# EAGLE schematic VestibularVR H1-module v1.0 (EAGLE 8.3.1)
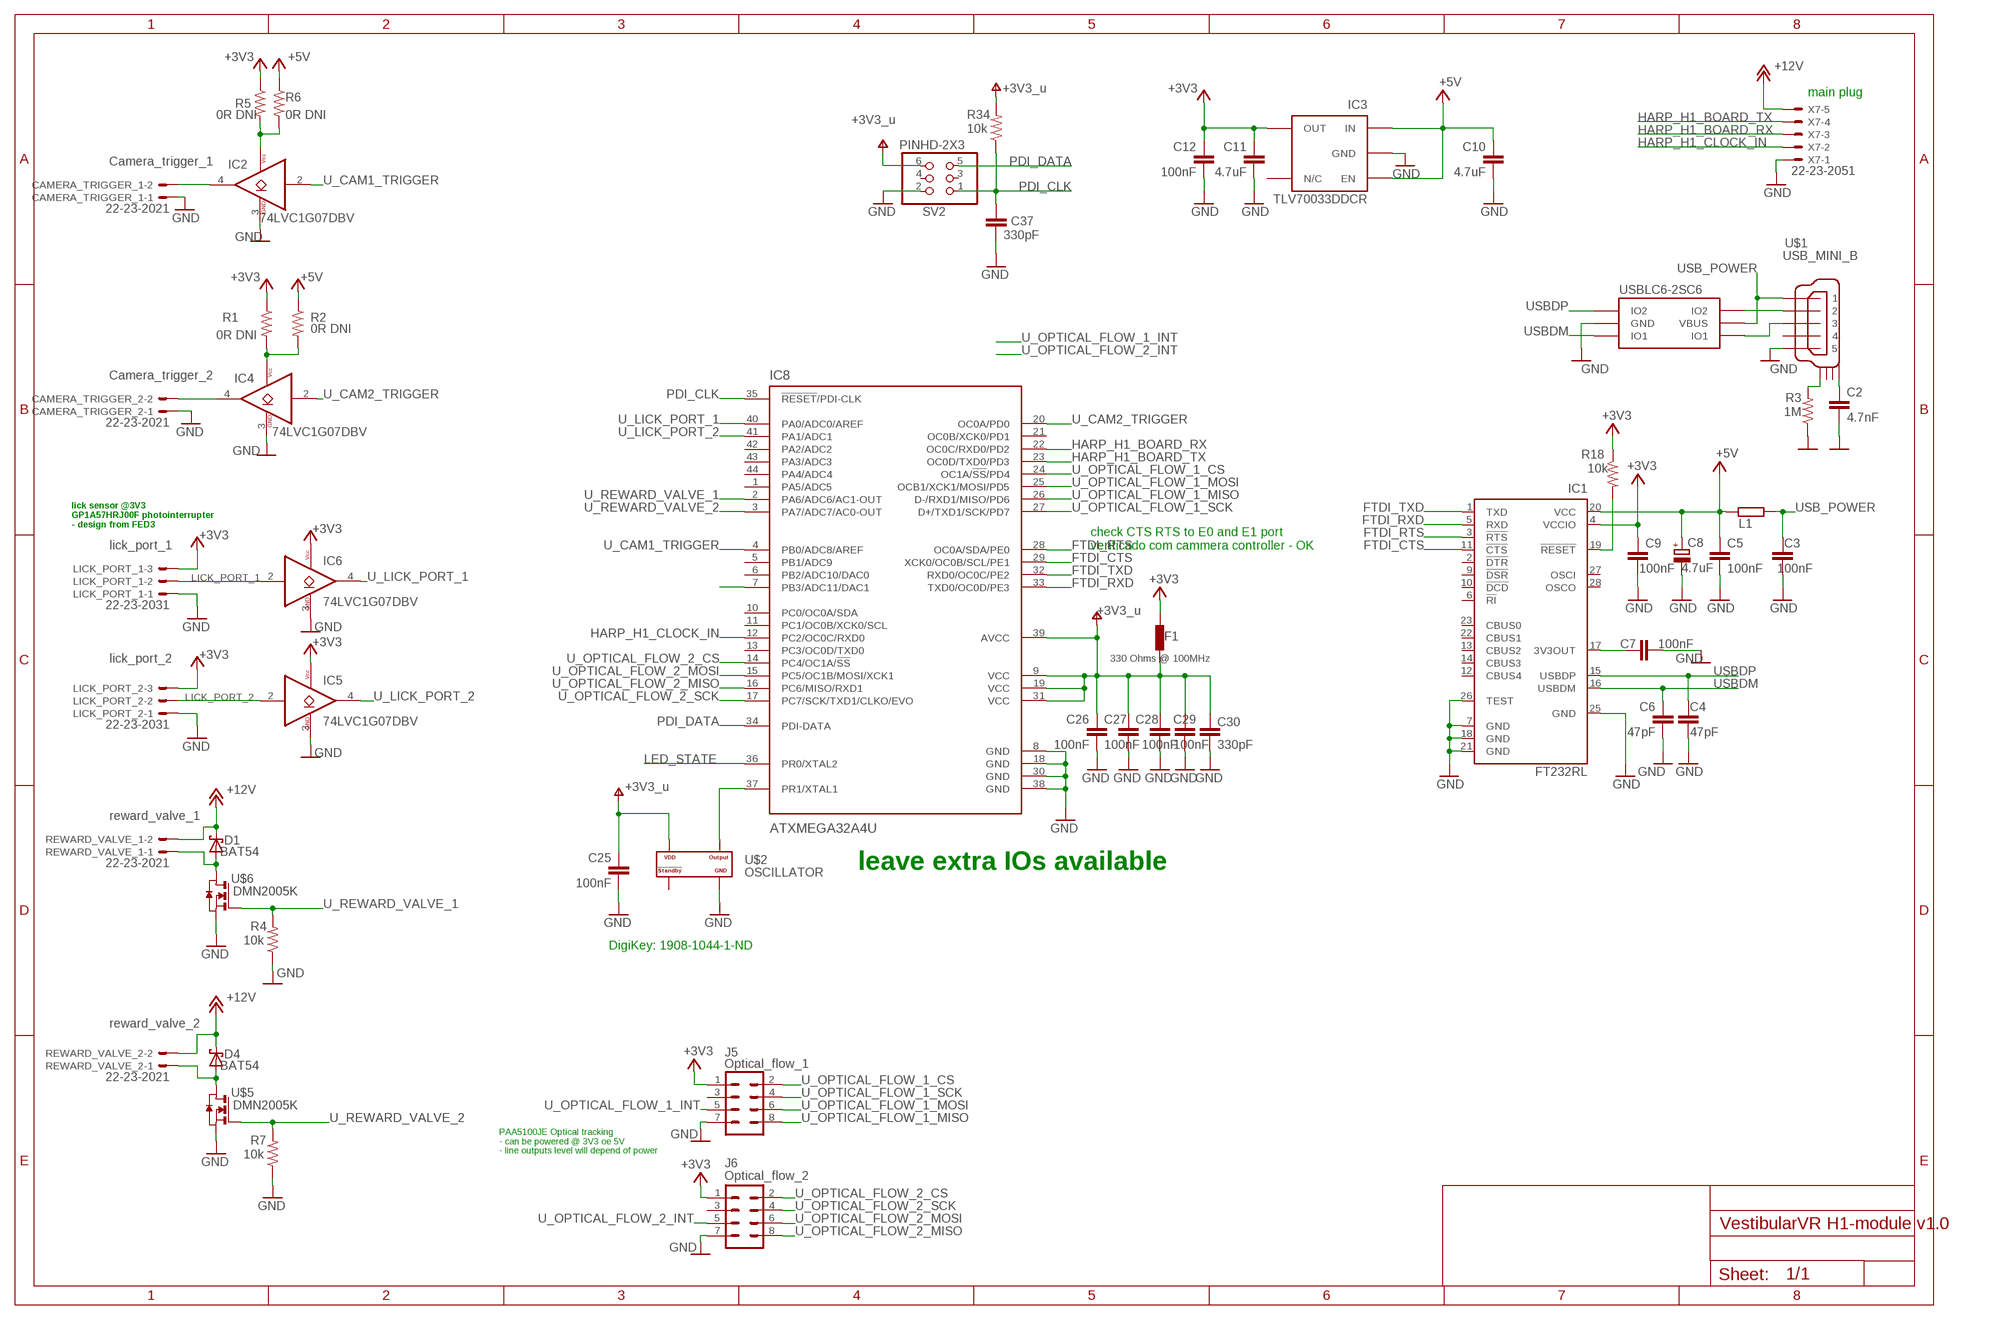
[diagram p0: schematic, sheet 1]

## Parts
C2  4.7nF  C-EUC0402  [C0402]
C3  100nF  C-EUC0402  [C0402]
C4  47pF  C-EUC0402  [C0402]
C5  100nF  C-EUC0402  [C0402]
C6  47pF  C-EUC0402  [C0402]
C7  100nF  C-EUC0402  [C0402]
C8  4.7uF  CPOL-EUA/3216-18R  [A/3216-18R]
C9  100nF  C-EUC0402  [C0402]
C10  4.7uF  C-EUC0603  [C0603]
C11  4.7uF  C-EUC0603  [C0603]
C12  100nF  C-EUC0402  [C0402]
C25  100nF  C-EUC0402  [C0402]
C26  100nF  C-EUC0402  [C0402]
C27  100nF  C-EUC0402  [C0402]
C28  100nF  C-EUC0402  [C0402]
C29  100nF  C-EUC0402  [C0402]
C30  330pF  C-EUC0402  [C0402]
C37  330pF  C-EUC0402  [C0402]
CAMERA_TRIGGER_1  22-23-2021  [22-23-2021]
CAMERA_TRIGGER_2  22-23-2021  [22-23-2021]
D1  BAT54  [SOT23]
D4  BAT54  [SOT23]
F1  330 Ohms @ 100MHz  BLM15HF0603  [R0603]
IC1  FT232RL  [SSOP28]
IC2  74LVC1G07DBV  [SOT23-5]
IC3  TLV70033DDCR  TLV700XX  [TSOT23-5]
IC4  74LVC1G07DBV  [SOT23-5]
IC5  74LVC1G07DBV  [SOT23-5]
IC6  74LVC1G07DBV  [SOT23-5]
IC7  USBLC6-2SC6  [SOT23-6L]
IC8  ATXMEGA32A4U  XMEGA-A4_AT-XMEGA-XXA4-AUTQFP44  [TQFP44]
J5  Optical_flow_1  CONN_04X2  [2X4]
J6  Optical_flow_2  CONN_04X2  [2X4]
L1  40R@100MHz  R-EU_R0805  [R0805]
LICK_PORT_1  22-23-2031  [22-23-2031]
LICK_PORT_2  22-23-2031  [22-23-2031]
R1  0R DNI  R-US_R0402  [R0402]
R2  0R DNI  R-US_R0402  [R0402]
R3  1M  R-US_R0402  [R0402]
R4  10k  R-US_R0402  [R0402]
R5  0R DNI  R-US_R0402  [R0402]
R6  0R DNI  R-US_R0402  [R0402]
R7  10k  R-US_R0402  [R0402]
R18  10k  R-US_R0402  [R0402]
R34  10k  R-US_R0402  [R0402]
REWARD_VALVE_1  22-23-2021  [22-23-2021]
REWARD_VALVE_2  22-23-2021  [22-23-2021]
SV2  PINHD-2X3  [2X03]
U$1  USB_MINI_B  [240-0002-1]
U$2  OSCILLATOR  [OSCILLATOR_3.2X2.5]
U$5  DMN2005K  [SOT23]
U$6  DMN2005K  [SOT23]
X7  22-23-2051  [22-23-2051]

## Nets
+3V3: C9.1 C11.1 C12.1 F1.2 IC1.4(VCCIO) IC3.5(OUT) IC5.5(VCC) IC6.5(VCC) J5.1 J6.1 LICK_PORT_1.3 LICK_PORT_2.3 R1.1 R5.1 R18.1
+3V3_U: C25.1 C26.1 C27.1 C28.1 C29.1 C30.1 F1.1 IC8.9(VCC) IC8.19(VCC) IC8.31(VCC) IC8.39(AVCC) R34.2 SV2.6 U$2.P$4(VDD) ; supply symbol labelled +3V3_u
+5V: C5.1 C8.+ C10.1 IC1.20(VCC) IC3.1(IN) IC3.3(EN) L1.1 R2.1 R6.1
+12V: X7.5
FTDI_CTS: IC1.11(!CTS) IC8.29(XCK0/OC0B/SCL/PE1)
FTDI_RTS: IC1.3(!RTS) IC8.28(OC0A/SDA/PE0)
FTDI_RXD: IC1.5(RXD) IC8.33(TXD0/OC0D/PE3)
FTDI_TXD: IC1.1(TXD) IC8.32(RXD0/OC0C/PE2)
GND: C2.2 C3.2 C4.2 C5.2 C6.2 C7.2 C8.- C9.2 C10.2 C11.2 C12.2 C25.2 C26.2 C27.2 C28.2 C29.2 C30.2 C37.2 CAMERA_TRIGGER_1.1 CAMERA_TRIGGER_2.1 IC1.7(GND) IC1.18(GND) IC1.21(GND) IC1.25(GND) IC1.26(TEST) IC2.3(GND) IC3.2(GND) IC4.3(GND) IC5.3(GND) IC6.3(GND) IC7.P$2(GND) IC8.8(GND) IC8.18(GND) IC8.30(GND) IC8.38(GND) J5.7 J6.7 LICK_PORT_1.1 LICK_PORT_2.1 R3.1 R4.1 R7.1 SV2.2 U$1.P$5 U$2.P$2(GND) U$5.2(S) U$6.2(S) X7.1
HARP_H1_BOARD_RX: IC8.22(OC0C/RXD0/PD2) X7.3
HARP_H1_BOARD_TX: IC8.23(OC0D/TXD0/PD3) X7.4
HARP_H1_CLOCK_IN: IC8.12(PC2/OC0C/RXD0) X7.2
LED_STATE: IC8.36(PR0/XTAL2)
LICK_PORT_1: IC6.2(A) LICK_PORT_1.2
LICK_PORT_2: IC5.2(A) LICK_PORT_2.2
N$1: R3.2 U$1.SHIELD_1
N$2: IC7.P$4(IO2) U$1.P$2
N$3: IC7.P$6(IO1) U$1.P$3
N$4: CAMERA_TRIGGER_2.2 IC4.4(Y)
N$5: IC4.5(VCC) R1.2 R2.2
N$6: D4.1(A) REWARD_VALVE_2.1 U$5.3(D)
N$7: D4.3(C) REWARD_VALVE_2.2
N$8: D1.3(C) REWARD_VALVE_1.2
N$9: D1.1(A) REWARD_VALVE_1.1 U$6.3(D)
N$14: IC2.5(VCC) R5.2 R6.2
N$16: CAMERA_TRIGGER_1.2 IC2.4(Y)
N$38: C7.1 IC1.17(3V3OUT)
N$59: C2.1 U$1.SHIELD_4
N$175: IC1.19(!RESET) R18.2
OSC2: IC8.37(PR1/XTAL1) U$2.P$3(OUTPUT)
PDI_CLK: C37.1 IC8.35(!RESET!/PDI-CLK) R34.1 SV2.1
PDI_DATA: IC8.34(PDI-DATA) SV2.5
U_CAM1_TRIGGER: IC2.2(A) IC8.4(PB0/ADC8/AREF)
U_CAM2_TRIGGER: IC4.2(A) IC8.20(OC0A/PD0)
U_HARPH1CLOCKIN: IC8.7(PB3/ADC11/DAC1)
U_LICK_PORT_1: IC6.4(Y) IC8.40(PA0/ADC0/AREF)
U_LICK_PORT_2: IC5.4(Y) IC8.41(PA1/ADC1)
U_OPTICAL_FLOW_1_CS: IC8.24(OC1A/!SS!/PD4) J5.2
U_OPTICAL_FLOW_1_INT: J5.5
U_OPTICAL_FLOW_1_MISO: IC8.26(D-/RXD1/MISO/PD6) J5.8
U_OPTICAL_FLOW_1_MOSI: IC8.25(OCB1/XCK1/MOSI/PD5) J5.6
U_OPTICAL_FLOW_1_SCK: IC8.27(D+/TXD1/SCK/PD7) J5.4
U_OPTICAL_FLOW_2_CS: IC8.14(PC4/OC1A/!SS) J6.2
U_OPTICAL_FLOW_2_INT: J6.5
U_OPTICAL_FLOW_2_MISO: IC8.16(PC6/MISO/RXD1) J6.8
U_OPTICAL_FLOW_2_MOSI: IC8.15(PC5/OC1B/MOSI/XCK1) J6.6
U_OPTICAL_FLOW_2_SCK: IC8.17(PC7/SCK/TXD1/CLKO/EVO) J6.4
U_REWARD_VALVE_1: IC8.2(PA6/ADC6/AC1-OUT) R4.2 U$6.1(G)
U_REWARD_VALVE_2: IC8.3(PA7/ADC7/AC0-OUT) R7.2 U$5.1(G)
USB_POWER: C3.1 IC7.P$5(VBUS) L1.2 U$1.P$1
USBDM: C6.1 IC1.16(USBDM) IC7.P$1(IO1)
USBDP: C4.1 IC1.15(USBDP) IC7.P$3(IO2)
Unconnected: IC1.2(!DTR) IC1.6(!RI) IC1.9(!DSR) IC1.10(!DCD) IC1.12(CBUS4) IC1.13(CBUS2) IC1.14(CBUS3) IC1.22(CBUS1) IC1.23(CBUS0) IC1.27(OSCI) IC1.28(OSCO) IC2.1(NC) IC3.4(N/C) IC4.1(NC) IC5.1(NC) IC6.1(NC) IC8.1(PA5/ADC5) IC8.5(PB1/ADC9) IC8.6(PB2/ADC10/DAC0) IC8.10(PC0/OC0A/SDA) IC8.11(PC1/OC0B/XCK0/SCL) IC8.13(PC3/OC0D/TXD0) IC8.21(OC0B/XCK0/PD1) IC8.42(PA2/ADC2) IC8.43(PA3/ADC3) IC8.44(PA4/ADC4) J5.3 J6.3 SV2.3 SV2.4 U$1.P$4 U$1.SHIELD_2 U$1.SHIELD_3 U$2.P$1(STANDBY#)

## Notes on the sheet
- main plug
- Camera_trigger_1
- Camera_trigger_2
- lick sensor @3V3
  GP1A57HRJ00F photointerrupter
  - design from FED3
- lick_port_1
- check CTS RTS to E0 and E1 port
  verificado com cammera controller - OK
- lick_port_2
- reward_valve_1
- leave extra IOs available
- DigiKey: 1908-1044-1-ND
- reward_valve_2
- PAA5100JE Optical tracking
  - can be powered @ 3V3 oe 5V
  - line outputs level will depend of power

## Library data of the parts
C2 = rcl:C-EU: CAPACITOR, European symbol; MPN: 04025C472KAT2A; SPICEPREFIX: C
C3 C5 C7 C9 = rcl:C-EU: CAPACITOR, European symbol; MPN: MC0402B104K160CT; SPICEPREFIX: C
C4 C6 = rcl:C-EU: CAPACITOR, European symbol; MPN: 04025A470JAT2A; SPICEPREFIX: C
C8 = rcl:CPOL-EU: POLARIZED CAPACITOR, European symbol; MPN: TAJA475K010; SPICEPREFIX: C
C10 C11 = rcl:C-EU: CAPACITOR, European symbol; MPN: C1608X6S1C475K080AC; NOTES: -; SPICEPREFIX: C; TYPE: SMD
C12 = rcl:C-EU: CAPACITOR, European symbol; MPN: MC0402B104K160CT; NOTES: -; SPICEPREFIX: C; TYPE: SMD
C25-C29 = rcl:C-EU: CAPACITOR, European symbol; DIGIKEY_PN: 445-5932-1-ND; MPN: C1005X7R1H104K050BB; NOTES: -; SPICEPREFIX: C; TYPE: SMD
C30 C37 = rcl:C-EU: CAPACITOR, European symbol; DIGIKEY_PN: 399-7787-1-ND; MPN: C0402C331J5GACTU; NOTES: -; SPICEPREFIX: C; TYPE: SMD
CAMERA_TRIGGER_1 CAMERA_TRIGGER_2 REWARD_VALVE_1 REWARD_VALVE_2 = con-molex:22-23-2021: .100" (2.54mm) Center Header - 2 Pin; MF: MOLEX; MPN: 22-23-2021; OC_FARNELL: 1462926; OC_NEWARK: 25C3832
D1 D4 = diode:BAT54: Schottky Diodes
F1 = VestibularVR H1-module v1.0:BLM15H: EMIFIL (R) Chip Ferrite Bead for GHz Noise; DIGIKEY_PN: 490-3997-1-ND; MOUSER_PN: 81-BLM18SG331TN1D; MPN: BLM18SG331TN1D; NOTES: -; TYPE: SMD
IC1 = VestibularVR H1-module v1.0:FT232R: UART/FIFO IC
IC2 IC4-IC6 = VestibularVR H1-module v1.0:74LVC1G07: Single Buffer/Driver With Open-Drain Output
IC3 = VestibularVR H1-module v1.0:TLV700XX: C REG LINEAR 3.3V 200MA SOT23-5; MPN: TLV70033DDCR; NOTES: -; TYPE: SMD
IC7 = VestibularVR H1-module v1.0:USBLC6-2SC6: TVS DIODE 5.25VWM 17VC SOT23-6
IC8 = VestibularVR H1-module v1.0:XMEGA-A4_AT-XMEGA-XXA4-AU: ATxMega a4 Serie; DIGIKEY_PN: ATXMEGA32A4U-AURCT-ND; MOUSER_PN: 556-ATXMEGA32A4U-AU; MPN: ATXMEGA32A4U-AUR
J5 J6 = SparkFun-Connectors:CONN_04X2: Multi connection point. Often used as Generic Header-pin footprint for 0.1 inch spaced/style header connections On any of the 0.1 inch spaced packages, you can populate with these: Break Away Headers - Straight (PRT-00116) Break Away Male Headers - Right Angle (PRT-00553) Female Headers (PRT-00115)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
L1 = rcl:R-EU_: RESISTOR, European symbol; MPN: MI0805K400R-10; SPICEPREFIX: R
LICK_PORT_1 LICK_PORT_2 = con-molex:22-23-2031: .100" (2.54mm) Center Header - 3 Pin; MF: MOLEX; MPN: 22-23-2031; OC_FARNELL: 1462950; OC_NEWARK: 30C0862
R1 R2 R5 R6 = rcl:R-US_: RESISTOR, American symbol; SPICEPREFIX: R
R3 = rcl:R-US_: RESISTOR, American symbol; PN: CRCW04021M00FKED; SPICEPREFIX: R
R4 R7 R34 = rcl:R-US_: RESISTOR, American symbol; DIGIKEY_PN: 541-3959-1-ND; MPN: CRCW040210K0FKED; NOTES: -; SPICEPREFIX: R; TYPE: SMD
R18 = rcl:R-US_: RESISTOR, American symbol; MPN: CRCW040210K0FKED; SPICEPREFIX: R
SV2 = Connector:PINHD-2X3: PIN HEADER; CATEGORY: CONNECTOR; SUB-CATEGORY: PIN-HEADER
U$1 = VestibularVR H1-module v1.0:USB_MINI_B: CONN RCPT USB2.0 MINI B SMD R/A
U$2 = VestibularVR H1-module v1.0:OSCILLATOR: XTAL OSC TCXO 32.0000MHZ HCMOS
U$5 U$6 = VestibularVR H1-module v1.0:DMN2005K: N-CHANNEL ENHANCEMENT MODE FIELD EFFECT TRANSISTOR
X7 = con-molex:22-23-2051: .100" (2.54mm) Center Header - 5 Pin; MF: MOLEX; MPN: 22-23-2051; OC_FARNELL: 1462952; OC_NEWARK: 38C9178

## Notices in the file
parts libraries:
SparkFun-Connectors: Licensing: Creative Commons ShareAlike 4.0 International - https://creativecommons.org/licenses/by-sa/4.0
